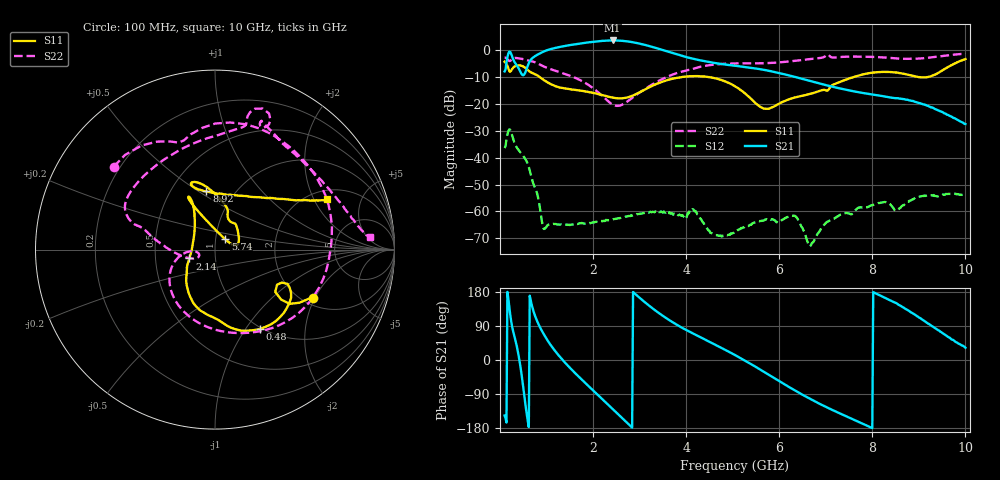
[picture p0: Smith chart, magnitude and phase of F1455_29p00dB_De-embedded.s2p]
! Integrated Device Technology
! Corporate Headquarters
! 6024 Silver Creek Valley Road
! San Jose, CA 95138  USA
! Phone:  1-408-284-8200
! Toll Free:  1-800-223-1366
! Webpage:  http://www.idt.com/
! Timing and RF Division
! 515 Groton Road, Suite 102
! Westford, MA 01886-6024
! Device:  F1455
! Description: 6-bit 0.5 dB Transmit Variable Gain Amplifier
! Frequency:  1400.0 -  2300.00 MHz
! Package:  6x6 mm Thin QFN Plastic Package: 28 pin
! State:  58
! Atten State:  29.0 dB
! Voltage:  +5.00 Volts
! Current:  217.646 mA
! Data:  The device was measured on a the F1455 evaluation board which has
!  individual transmission lines to the RF pins.  Data was collected
!  using a calibrated network analyzer.  The evaluation board was
!  de-embedded using a TRL calibration technique.
!  The reference plane is the edge of the package pin.
!  Pin  1 = CSb
!  Pin  2 = DATA
!  Pin  3 = CLK
!  Pin  4 = RSET
!  Pin  5 = GND
!  Pin  6 = RFIN  = Port 1
!  Pin  7 = GND
!  Pin  8 = NC
!  Pin  9 = NC
!  Pin 10 = NC
!  Pin 11 = NC
!  Pin 12 = NC
!  Pin 13 = NC
!  Pin 14 = /STBY
!  Pin 15 = GND
!  Pin 16 = RFOUT  = Port 2
!  Pin 17 = GND
!  Pin 18 = NC
!  Pin 19 = NC
!  Pin 20 = NC
!  Pin 21 = GND
!  Pin 22 = NC
!  Pin 23 = GND
!  Pin 24 = NC
!  Pin 25 = NC
!  Pin 26 = NC
!  Pin 27 = GND
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# GHz S dB R 50
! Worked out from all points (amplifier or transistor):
!   496 points, 100 MHz to 10 GHz, reference 50 ohm
!   highest |S21| = 3.6 dB at 2.42 GHz (marker M1)
!   |S21| within 3 dB of that: 1.139 GHz to 3.391 GHz (2.252 GHz wide, 99.4 % of centre)
!   unconditionally stable (mu >= 1): start of sweep to end of sweep
!   at 1.74 GHz: K = 553.33, MAG = 3.0 dB, |S12| = -64.4 dB
!   at 5.06 GHz: K = 1520.37, MAG = -3.9 dB, |S12| = -67.7 dB
!   at 10 GHz: K = 780.28, MAG = -18.8 dB, |S12| = -53.8 dB
!   S11 on the Smith chart (normalised r, x): 100 MHz: 2.27, -1.95; 480 MHz: 0.98, -1.17; 2.14 GHz: 0.75, -0.08; 5.74 GHz: 1.11, +0.13; 8.92 GHz: 0.74, +0.54; 10 GHz: 2.43, +2.56
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0.1  -4.28 -26.1  -7.88 -146.5  -36.40 47.9  -2.74 140.7
0.18  -6.70 -37.1  -1.22 161.6  -30.07 -6.2  -3.72 112.4
0.26  -7.00 -25.3  -2.23 89.0  -31.59 -77.4  -3.33 96.1
0.38  -5.66 -42.7  -6.09 25.6  -36.67 -119.0  -2.97 58.2
0.48  -5.88 -60.6  -9.15 -52.6  -38.92 -150.6  -3.23 31.4
0.66  -8.18 -87.9  -3.60 157.5  -46.18 140.0  -4.01 -10.8
0.78  -9.11 -103.1  -1.90 108.0  -52.33 115.7  -4.66 -37.5
0.96  -11.29 -123.6  -0.32 64.2  -66.47 130.2  -6.18 -71.2
1.34  -14.04 -142.3  1.42 1.0  -65.00 121.3  -8.49 -121.0
1.76  -15.10 -151.2  2.61 -52.1  -64.29 92.1  -11.44 -156.1
2.14  -16.45 -161.0  3.40 -96.5  -63.74 79.0  -16.09 -174.9
2.42  -17.63 -177.0  3.65 -129.4  -62.95 70.6  -20.21 -170.2
2.84  -16.95 145.1  3.03 -178.3  -61.56 58.7  -17.75 -157.3
3.4  -12.30 118.6  0.59 125.2  -59.89 36.2  -11.53 178.2
4.1  -9.65 116.2  -2.97 72.9  -59.31 16.0  -7.14 163.0
5.06  -13.50 111.9  -5.80 12.4  -67.66 40.5  -4.90 148.1
5.74  -21.81 44.9  -7.51 -36.4  -62.90 32.6  -4.79 120.0
6.34  -17.56 13.9  -9.94 -80.5  -61.68 -10.6  -3.95 89.5
6.7  -16.08 34.3  -11.62 -105.0  -71.79 -172.7  -3.22 78.6
8.36  -8.08 109.5  -17.51 158.7  -56.88 64.2  -2.83 62.6
8.92  -9.68 98.4  -19.21 119.3  -54.85 77.1  -3.15 40.2
10  -3.28 24.1  -27.47 32.4  -53.83 9.7  -1.27 4.7
